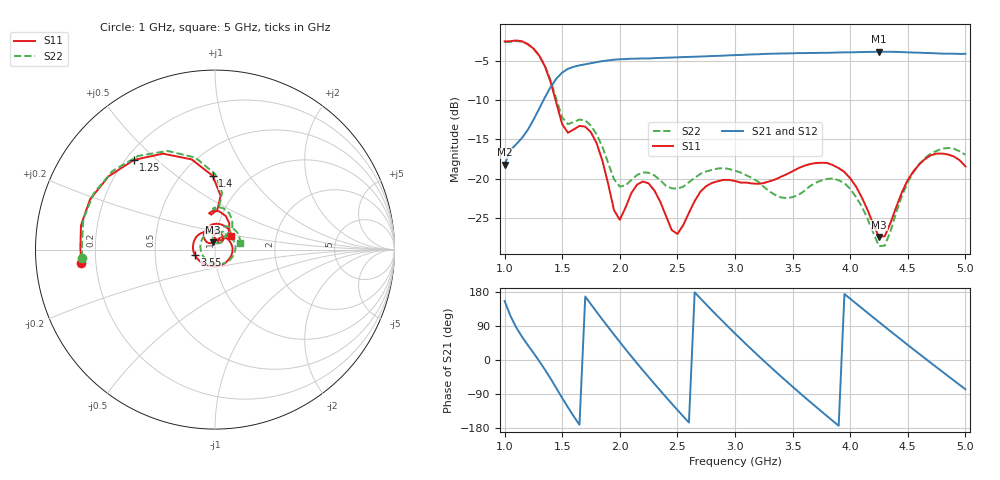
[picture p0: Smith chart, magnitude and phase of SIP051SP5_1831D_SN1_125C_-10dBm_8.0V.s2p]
# GHz  S  dB  R  50
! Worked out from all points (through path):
!   81 points, 1 GHz to 5 GHz, reference 50 ohm
!   highest |S21| = -3.84 dB at 4.25 GHz (marker M1); lowest = -18.2 dB at 1 GHz (marker M2)
!   lowest |S11| = -27.4 dB at 4.25 GHz (marker M3), VSWR 1.09, Z = 48.5 + j3.92 ohm
!   |S11| at or under -10 dB: 1.442 GHz to end of sweep
!   |S22| runs from -28.6 to -2.5 dB; largest |S21 - S12| = 0.0016
!   S11 on the Smith chart (normalised r, x): 1 GHz: 0.14, -0.05; 1.25 GHz: 0.23, +0.42; 1.4 GHz: 0.70, +0.69; 3.55 GHz: 0.80, -0.05; 5 GHz: 1.18, +0.19
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1  -2.52 -174.3  -18.21 155.7  -18.20 155.7  -2.59 -176.3
1.25  -3.43 132.2  -12.52 19.0  -12.53 18.9  -3.41 129.4
1.4  -7.72 91.8  -8.32 -49.6  -8.31 -49.6  -7.51 90.0
1.55  -14.16 96.1  -6.01 -125.0  -6.00 -125.0  -13.06 91.4
1.7  -13.38 83.6  -5.43 167.6  -5.42 167.6  -12.58 78.6
1.9  -20.74 47.9  -4.94 86.5  -4.92 86.5  -18.06 49.9
2  -25.24 78.7  -4.79 47.5  -4.78 47.6  -21.01 62.3
2.1  -21.86 94.2  -4.72 9.6  -4.72 9.8  -20.17 72.7
2.2  -20.37 76.5  -4.68 -27.0  -4.69 -27.0  -19.20 64.9
2.35  -22.90 50.5  -4.62 -80.3  -4.62 -80.2  -20.19 52.0
2.5  -27.05 63.8  -4.55 -131.8  -4.54 -131.8  -21.29 52.2
2.65  -22.85 67.2  -4.47 178.6  -4.46 178.6  -19.91 48.9
2.85  -20.33 20.2  -4.36 115.4  -4.36 115.4  -18.72 23.3
3  -20.30 -23.0  -4.27 70.0  -4.26 70.0  -18.99 -2.9
3.25  -20.56 -95.8  -4.12 -2.2  -4.11 -2.1  -21.05 -62.0
3.55  -18.67 -165.2  -4.01 -83.8  -4.02 -83.8  -22.09 -172.7
3.7  -18.02 163.5  -3.99 -122.8  -3.98 -122.8  -20.53 137.3
3.95  -19.15 115.5  -3.91 174.1  -3.91 174.2  -20.57 76.9
4.25  -27.42 108.5  -3.84 100.2  -3.83 100.2  -28.60 66.5
4.35  -25.63 135.3  -3.85 75.8  -3.85 75.9  -26.71 98.1
4.65  -17.50 105.4  -3.99 4.2  -4.00 4.2  -17.37 72.2
5  -18.43 40.9  -4.10 -77.2  -4.11 -77.3  -16.96 14.0
